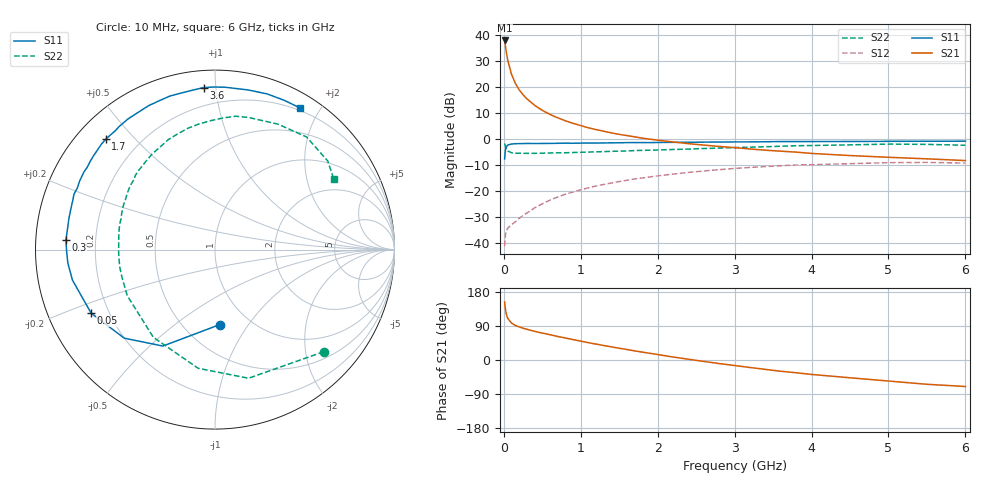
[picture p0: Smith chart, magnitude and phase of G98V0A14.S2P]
! SIEMENS Small Signal Semiconductors
! BFG235
! Si NPN RF Bipolar Junction Transistor in SOT223
! VCE = 8 V  IC = 140 mA
! Common Emitter S-Parameters:  July  1994
# GHz  S  MA  R  50
!  f  S11  S21  S12  S22
! GHz  MAG  ANG  MAG  ANG  MAG  ANG  MAG  ANG
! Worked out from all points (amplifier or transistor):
!   40 points, 10 MHz to 6 GHz, reference 50 ohm
!   highest |S21| = 38.0 dB at 10 MHz (marker M1)
!   |S21| within 3 dB of that: start of sweep to 24.9 MHz
!   unconditionally stable (mu >= 1): 462.2 MHz to 1.45 GHz
!   at 200 MHz: K = 0.80, MSG = 24.7 dB, |S12| = -30.4 dB
!   at 1.5 GHz: K = 1.00, MSG = 9.1 dB, |S12| = -16.2 dB
!   at 6 GHz: K = 0.88, MSG = 0.5 dB, |S12| = -9.1 dB
!   S11 on the Smith chart (normalised r, x): 10 MHz: 0.74, -0.75; 50 MHz: 0.13, -0.24; 300 MHz: 0.09, +0.03; 1.7 GHz: 0.08, +0.41; 3.6 GHz: 0.09, +0.93; 6 GHz: 0.17, +1.75
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0.01  0.4185 -86.2  79.7 153.2  0.0088 63.6  0.8311 -43.2
0.02  0.6108 -118.4  63.39 134.4  0.0142 49.3  0.7407 -75.4
0.03  0.7065 -135.7  49.98 122.6  0.0169 41.3  0.6678 -98.1
0.05  0.7755 -152.8  33.46 109.8  0.0195 34.4  0.5973 -125.1
0.1  0.8122 -167.9  17.73 97.4  0.0229 36.7  0.5522 -152.3
0.15  0.8231 -174.7  11.93 91.2  0.0259 42.3  0.5408 -163.7
0.2  0.8257 -178.3  8.93 87.3  0.0301 47.3  0.5396 -170.0
0.25  0.8289 178.7  7.186 83.8  0.0342 50.6  0.5369 -174.4
0.3  0.8323 176.2  6 81.1  0.0382 53.2  0.537 -178.1
0.4  0.8299 171.7  4.515 75.7  0.0479 56.4  0.5373 176.7
0.5  0.8322 168.0  3.602 71.0  0.0575 57.8  0.5409 172.5
0.6  0.834 164.8  3.01 66.8  0.0676 57.8  0.5453 168.6
0.8  0.8441 158.6  2.271 58.1  0.0877 56.2  0.551 161.9
1.1  0.8486 149.4  1.665 45.6  0.1166 51.7  0.5689 152.9
1.4  0.8551 142.2  1.329 34.6  0.1447 45.9  0.5873 144.6
1.7  0.8656 134.8  1.115 24.0  0.1726 39.6  0.6068 136.9
2.2  0.8745 123.6  0.891 7.9  0.2142 28.6  0.6377 123.3
3.2  0.8923 102.2  0.652 -19.8  0.2874 5.6  0.7051 97.4
3.6  0.9052 94.0  0.591 -29.7  0.31 -4.4  0.7354 86.3
4.5  0.9085 78.3  0.487 -46.9  0.3398 -24.3  0.7819 63.4
5.5  0.9171 65.0  0.421 -64.1  0.3591 -46.2  0.7988 38.1
6  0.9202 59.1  0.39 -69.9  0.3496 -54.6  0.769 30.6
